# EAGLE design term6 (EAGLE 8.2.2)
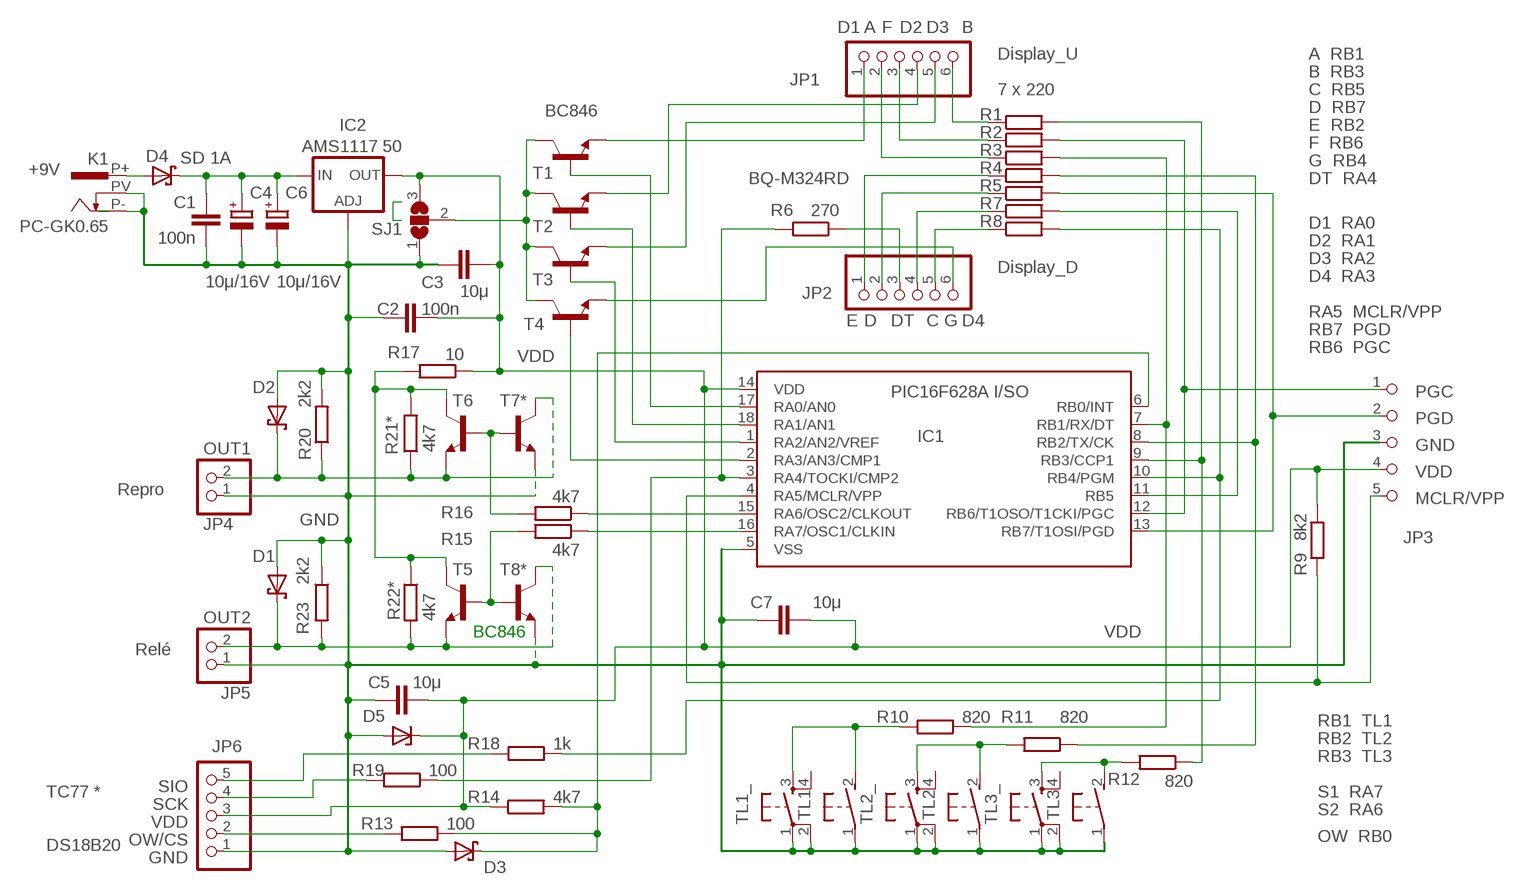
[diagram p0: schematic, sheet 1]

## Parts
C1  100n  C-EUC0805  [C0805]
C2  100n  C-EUC1206  [C1206]
C3  10μ  C-EUC1206  [C1206]
C4  10μ/16V  CPOL-EUSMCC  [SMC_C]
C5  10μ  C-EUC0805  [C0805]
C6  10μ/16V  CPOL-EUSMCD  [SMC_D]
C7  10μ  C-EUC1206  [C1206]
D1  ESD5V0S1U-02V  [SUPRES_D]
D2  ESD5V0S1U-02V  [SUPRES_D]
D3  ESD5V0S1U-02V  [SUPRES_D]
D4  SD 1A  SDIODE-1A  [SOD-5]
D5  ZENER-DIODESOD80C  [SOD80C]
IC1  PIC16F628A I/SO  PIC16F628SO  [SO-18W]
IC2  AMS1117 50  LD117AS12TR  [SOT223]
JP1  PINHD-1X061X06G  [1X06G]
JP2  PINHD-1X061X06G  [1X06G]
JP3  PIN5  [PIN5]
JP4  OUT1  PINHD-1X02_2.54-S  [1X02-S]
JP5  OUT2  PINHD-1X02_2.54-S  [1X02-S]
JP6  PINHD-1X05_2.54-S  [1X05-S]
K1  PC-GK0.65  [PC-GK0.65]
R1  R-EU_R0805  [R0805]
R2  R-EU_R0805  [R0805]
R3  R-EU_R0805  [R0805]
R4  R-EU_R0805  [R0805]
R5  R-EU_R0805  [R0805]
R6  270  R-EU_R0805  [R0805]
R7  R-EU_R0805  [R0805]
R8  R-EU_R0805  [R0805]
R9  8k2  R-EU_R0805  [R0805]
R10  820  R-EU_R0805  [R0805]
R11  820  R-EU_R0805  [R0805]
R12  820  R-EU_R0805  [R0805]
R13  100  R-EU_R0805  [R0805]
R14  4k7  R-EU_R0805  [R0805]
R15  4k7  R-EU_R0805  [R0805]
R16  4k7  R-EU_R0805  [R0805]
R17  10  R-EU_R0805  [R0805]
R18  1k  R-EU_R0805  [R0805]
R19  100  R-EU_R0805  [R0805]
R20  2k2  R-EU_R0805  [R0805]
R21*  4k7  R-EU_R0805  [R0805]
R22*  4k7  R-EU_R0805  [R0805]
R23  2k2  R-EU_R0805  [R0805]
SJ1  SJ2W  [SJ_2]
T1  BC846ASMD  [SOT23]
T2  BC817-16SMD  [SOT23-BEC]
T3  BC817-16SMD  [SOT23-BEC]
T4  BC846  BC817-16SMD  [SOT23-BEC]
T5  BC846  BC817-16SMD  [SOT23-BEC]
T6  BC846  BC817-16SMD  [SOT23-BEC]
T7*  BC846  BC817-16SMD  [SOT23-BEC]
T8*  BC846  BC817-16SMD  [SOT23-BEC]
TL1  DTSM-3  [DTSM-3]
TL1_  T_SWITCH  [T_SWITCH]
TL2  DTSM-3  [DTSM-3]
TL2_  T_SWITCH  [T_SWITCH]
TL3  DTSM-3  [DTSM-3]
TL3_  T_SWITCH  [T_SWITCH]

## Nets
A: JP1.2 R3.1
B: JP1.6 R1.1
C: JP2.4 R7.1
D: JP2.2 R5.1
D1: JP1.1 T1.2(E)
D2: JP1.4 T2.E
D3: JP1.5 T3.E
D4: JP2.6 T4.E
DT: JP2.3 R6.1
E: JP2.1 R4.1
F: JP1.3 R2.1
G: JP2.5 R8.1
GND: C1.1 C2.2 C3.2 C4.- C5.2 C6.- C7.2 D1.A D2.A D3.A D5.A IC1.5(VSS) IC2.1(ADJ) JP3.3(_3) JP4.1 JP5.1 JP6.1 K1.P- K1.PV R20.2 R23.1 SJ1.1 T7*.E T8*.E TL1.1 TL1_.1 TL1_.2 TL2.1 TL2_.1 TL2_.2 TL3.1 TL3_.1 TL3_.2
MCLR/VPP: IC1.4(RA5/MCLR/VPP) JP3.5(_5) R9.2
N$1: JP6.4 R19.2
N$2: R15.2 T5.B T8*.B
N$4: IC1.17(RA0/AN0) T1.1(B)
N$5: IC1.18(RA1/AN1) T2.B
N$6: IC1.1(RA2/AN2/VREF) T3.B
N$7: IC1.2(RA3/AN3/CMP1) T4.B
N$8: R12.2 TL3.2 TL3_.3
N$9: D1.C JP5.2 R22*.2 R23.2 T5.E T8*.C
N$10: D4.A K1.P+
N$11: D3.C IC1.6(RB0/INT) R13.1 R14.2
N$12: R16.2 T6.B T7*.B
N$13: R17.2 R21*.2 R22*.1 T5.C T6.C
N$14: JP6.5 R18.2
N$15: SJ1.2 T1.3(C) T2.C T3.C T4.C
N$17: IC1.8(RB2/TX/CK) R4.2 R11.1
N$19: IC1.11(RB5) R7.2
N$20: IC1.10(RB4/PGM) R8.2 R18.1
N$21: IC1.9(RB3/CCP1) R1.2 R12.1
N$22: IC1.3(RA4/TOCKI/CMP2) R6.2 R19.1
N$23: IC1.7(RB1/RX/DT) R3.2 R10.1
N$25: C1.2 C4.+ C6.+ D4.C IC2.3(IN)
N$28: R11.2 TL2.2 TL2_.3
N$29: R10.2 TL1.2 TL1_.3
N$34: IC1.16(RA7/OSC1/CLKIN) R15.1
N$35: IC1.15(RA6/OSC2/CLKOUT) R16.1
OW/CS: JP6.2 R13.2
PGC: IC1.12(RB6/T1OSO/T1CKI/PGC) JP3.1(_1) R2.2
PGD: IC1.13(RB7/T1OSI/PGD) JP3.2(_2) R5.2
S2: D2.C JP4.2 R20.1 R21*.1 T6.E T7*.C
VDD: C2.1 C3.1 C5.1 C7.1 D5.C IC1.14(VDD) IC2.2(OUT) IC2.4(OUT) JP3.4(_4) JP6.3 R9.1 R14.1 R17.1 SJ1.3
Unconnected: TL1_.4 TL2_.4 TL3_.4

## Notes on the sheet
- Display_U | A  RB1
- B  RB3
- 7 x 220 | C  RB5
- D  RB7
- E  RB2
- F  RB6
- G  RB4
- +9V
- BQ-M324RD | DT  RA4
- D1  RA0
- D2  RA1
- D3  RA2
- Display_D
- D4  RA3
- RA5  MCLR/VPP
- RB7  PGD
- RB6  PGC
- Repro
- JP3
- BC846
- Relé
- RB1  TL1
- RB2  TL2
- RB3  TL3
- SIO
- TC77 * | SCK | S1  RA7
- S2  RA6
- OW  RB0
- DS18B20

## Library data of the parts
C1-C3 C5 C7 = rcl:C-EU: CAPACITOR, European symbol
C4 C6 = rcl:CPOL-EU: POLARIZED CAPACITOR, European symbol
D1-D3 = pdk1:ESD5V0S1U-02V
D4 = pdk1:SDIODE-1A
D5 = diode:ZENER-DIODE: Z-Diode
IC1 = microchip:PIC16F62*: FLASH-Based 8-Bit CMOS Microcontroller Source: http://ww1.microchip.com/downloads/en/DeviceDoc/40300C.pdf; MF: MICROCHIP; MPN: PIC16F628-20I/SO; OC_FARNELL: 9760415; OC_NEWARK: 23C4986
IC2 = v-reg:LD117A?*: Low drop fixed and adjustable positive voltage regulators 1 A Source: http://www.st.com/stonline/products/literature/ds/7194/ld1117axx.pdf
JP1 JP2 = pinhead-2:PINHD-1X06: PIN HEADER
JP3 = pdk1:PIN5
JP4 JP5 = pinhead-2:PINHD-1X02: PIN HEADER
JP6 = pinhead-2:PINHD-1X05: PIN HEADER
K1 = pdk1:PC-GK0.65
R1-R20 R21* R22* R23 = rcl:R-EU_: RESISTOR, European symbol
SJ1 = jumper:SJ2W: SMD solder JUMPER
T1 = transistor-npn:BC846*: NPN Transistor
T2-T6 T7* T8* = transistor-npn:BC817*: NPN Transistor
TL1-TL3 = switch-tact_1:DTSM-3
TL1_ TL2_ TL3_ = pdk1:T_SWITCH

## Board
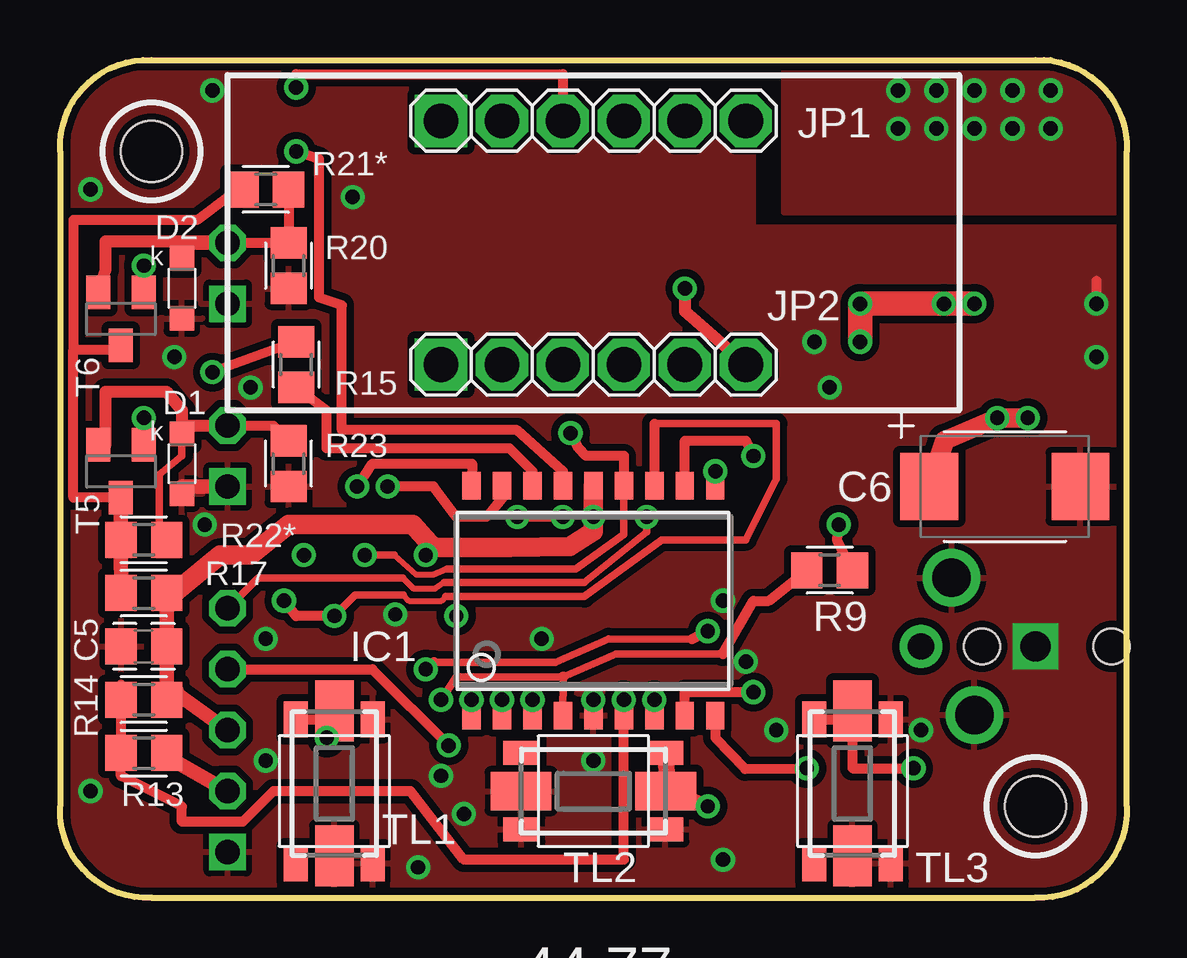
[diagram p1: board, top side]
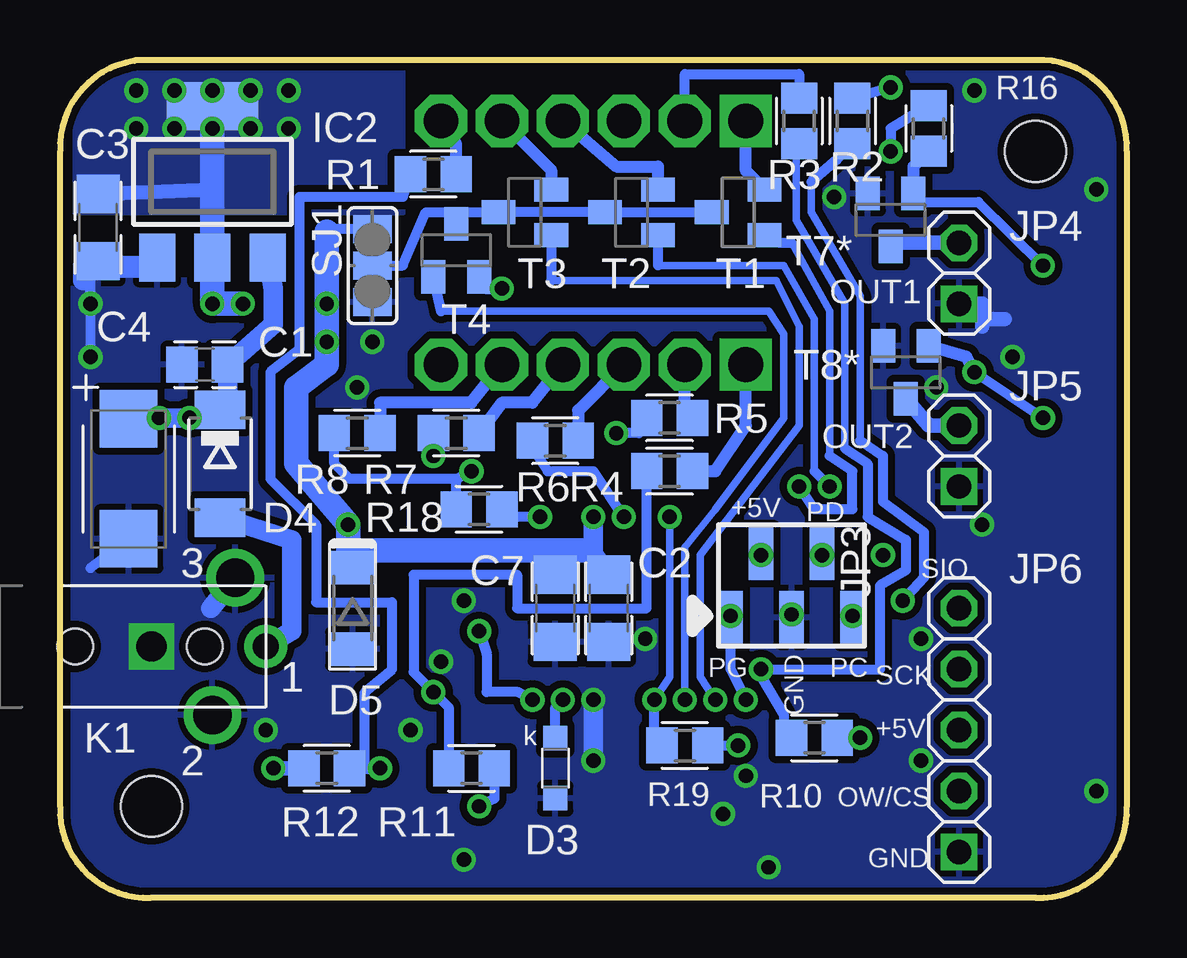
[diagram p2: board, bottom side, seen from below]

Size 44.45 x 34.92 mm. Coordinates in mm from the lower left corner, seen from the top.
Outline: 40.64,34.92 arc-95 44.45,31.11 44.45,3.81 arc-95 40.64,0 3.81,0 arc-95 0,3.81 0,31.11 arc-95 3.81,34.92 41.27,34.92
Copper layers (1*16): Top 0.035mm / dielectric 1.5mm / Bottom 0.035mm
Design rules "default *": minimum track width 6mil, minimum drill 0.35mm, track to track 6mil, track to pad 6mil, pad to pad 6mil, via to via 6mil, smd to smd 0mil, copper to edge 5mil, drill to drill 6mil, minimum pad ring 10mil, minimum via ring 8mil, stop-mask expansion 4mil, vias tented up to drill 0mil, thermal gap 10mil
Holes 2.54 mm at 40.64,3.81 3.81,31.11

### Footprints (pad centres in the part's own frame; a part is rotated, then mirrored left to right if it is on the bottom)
C0805 = smd 1.3 x 1.5: 1 -0.95,0; 2 0.95,0
C1206 = smd 1.6 x 1.8: 1 -1.4,0; 2 1.4,0
SMC_C = smd 2.4 x 2.4: + -2.5,0; - 2.5,0
SMC_D = smd 2.4 x 2.8: + -3.15,0; - 3.15,0
SUPRES_D = smd 1.016 x 1.016: A 1.25,0; C -1.25,0
SOD-5 = smd 1.6 x 2.1: A 2.25,0; C -2.25,0
SOD80C = smd 1.4 x 1.8: A 1.7,0; C -1.7,0
SO-18W = smd 0.762 x 1.143: 1 -5.08,-4.788; 2 -3.81,-4.788; 3 -2.54,-4.788; 4 -1.27,-4.788; 5 0,-4.788; 6 1.27,-4.788; 7 2.54,-4.788; 8 3.81,-4.788; 9 5.08,-4.788; 10 5.08,4.788; 11 3.81,4.788; 12 2.54,4.788; 13 1.27,4.788; 14 0,4.788; 15 -1.27,4.788; 16 -2.54,4.788; 17 -3.81,4.788; 18 -5.08,4.788
SOT223 = smd 1.5 x 2: 1 -2.3,-3.15; 2 0,-3.15; 3 2.3,-3.15 | smd 3.8 x 2: 4 0,3.15
1X06G = drill 1.448 pad 1.93 square: 1 -6.35,0 | drill 1.448 pad 1.93 octagon: 2 -3.81,0; 3 -1.27,0; 4 1.27,0; 5 3.81,0; 6 6.35,0
PIN5 = smd 1.016 x 2.2: 1 -1.905,1.33; 2 -0.635,-1.33; 3 0.635,1.33; 4 1.905,-1.33; 5 3.175,1.33
1X02-S = drill 1.016 square: 1 -1.27,0 | drill 1.016 octagon: 2 1.27,0
1X05-S = drill 1.016 square: 1 -5.08,0 | drill 1.016 octagon: 2 -2.54,0; 3 0,0; 4 2.54,0; 5 5.08,0
PC-GK0.65 = drill 1.1 pad 1.778: P+ -5.08,0 | drill 1.6: P- -2.857,2.857; PV -3.81,-2.857 | hole 1.5: -2.54,0; 2.857,0
R0805 = smd 1.3 x 1.5: 1 -0.95,0; 2 0.95,0
SJ_2 = smd 1.168 x 1.6: 1 -1.524,0; 2 0,0; 3 1.524,0
SOT23 = smd 1 x 1.4: 1 -0.95,-1.1; 2 0.95,-1.1; 3 0,1.1
SOT23-BEC = smd 1 x 1.4: B -0.95,-1.1; C 0,1.1; E 0.95,-1.1
DTSM-3 = smd 2.54 x 1.6: 1 -3.018,0; 2 3.018,0
T_SWITCH = smd 1.5 x 1: 1 -3,1.6; 2 3,1.6; 3 -3,-1.6; 4 3,-1.6

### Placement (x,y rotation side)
C1  38.42,22.23 0 bottom
C2  21.59,12.06 270 bottom
C3  42.86,27.94 270 bottom
C4  41.59,17.46 270 bottom
C5  3.49,10.48 180 top
C6  39.37,17.14 0 top
C7  23.81,12.06 270 bottom
D1  5.08,18.1 270 top
D2  5.08,25.4 270 top
D3  23.81,5.4 270 bottom
D4  37.78,18.1 270 bottom
D5  32.26,12.06 270 bottom
IC1  22.23,12.38 0 top
IC2  38.1,29.84 0 bottom
JP1  22.23,32.38 0 top
JP2  22.23,22.23 0 top
JP3  13.34,13.02 180 bottom
JP4  6.99,26.04 90 bottom
JP5  6.99,18.41 90 bottom
JP6  6.99,6.99 90 bottom
K1  40.96,10.48 180 bottom
R1  28.89,30.16 180 bottom
R2  11.43,32.38 270 bottom
R3  13.65,32.38 270 bottom
R4  19.05,17.78 180 bottom
R5  19.05,20 180 bottom
R6  23.81,19.05 180 bottom
R7  27.94,19.37 180 bottom
R8  32.07,19.37 180 bottom
R9  32.07,13.65 180 top
R10  13.02,6.67 0 bottom
R11  27.3,5.4 0 bottom
R12  33.34,5.4 180 bottom
R13  3.49,6.03 0 top
R14  3.49,8.26 180 top
R15  9.84,22.23 90 top
R16  8.26,32.07 270 bottom
R17  3.49,12.7 180 top
R18  26.99,16.19 0 bottom
R19  18.41,6.35 0 bottom
R20  9.53,26.35 270 top
R21*  8.57,29.53 180 top
R22*  3.49,14.92 0 top
R23  9.53,18.1 90 top
SJ1  31.43,26.35 90 bottom
T1  16.19,28.57 90 bottom
T2  20.64,28.57 90 bottom
T3  25.08,28.57 90 bottom
T4  27.94,26.99 0 bottom
T5  2.54,17.78 180 top
T6  2.54,24.13 180 top
T7*  9.84,28.26 180 bottom
T8*  9.21,21.91 180 bottom
TL1  11.43,4.76 90 top
TL1_  11.43,4.45 270 top
TL2  22.23,4.45 0 top
TL2_  22.23,4.45 180 top
TL3  33.02,4.76 90 top
TL3_  33.02,4.45 270 top

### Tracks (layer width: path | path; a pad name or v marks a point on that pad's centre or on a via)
A
  Bottom 0.406: JP1.2 18.41,34.34 13.65,34.34 R3.1
B
  Bottom 0.508: R1.1 27.94,31.43 JP1.6
C
  Bottom 0.508: JP2.4 24.77,20.64 26.04,20.64 R7.1
D
  Bottom 0.406: R5.1 18.41,20.32
  Bottom 0.508: 18.41,20.32 JP2.2
D1
  Bottom 0.508: T1.2 15.88,30.31 JP1.1
D2
  Bottom 0.508: JP1.4 21.27,30.48 19.54,30.48 T2.E
D3
  Bottom 0.508: JP1.5 23.98,30.33 T3.E
D4  (via drill 0.6)
  Top 0.508: JP2.6 26.04,24.45 v26.04,25.4
  Bottom 0.508: v26.04,25.4 26.67,25.4 T4.E
DT
  Bottom 0.406: 22.86,19.37 R6.1
  Bottom 0.508: JP2.3 22.86,20.32 22.86,19.37
E
  Bottom 0.508: R4.1 17.14,17.78 15.88,19.68 JP2.1
F  (via drill 0.6)
  Top 0.406: JP1.3 20.95,34.34 9.84,34.34 9.84,34.29 v9.84,33.78
  Bottom 0.406: R2.1 v9.84,33.78
G
  Bottom 0.406: R8.1
  Bottom 0.508: JP2.5 27.3,20.64 31.11,20.64 R8.1
GND  (via drill 0.6, 1.27)
  Top 0.406: 43.18,25.72 v43.18,24.77
  Top 0.61: JP5.1 5.1,17.14
  Bottom 0.406: IC2.1 40.4,26.04 43.18,26.04 v43.18,24.77 | v43.18,24.77 v43.18,22.54 | 43.18,13.74 C4.- | v43.18,24.77 43.18,26.36 C3.2
  Bottom 0.61: JP4.1 6.03,24.77 6.03,23.81 | 5.08,24.13 5.71,24.13
  Bottom 0.813: 42.55,26.35 40.32,26.35 | C3.2 42.55,26.35 | 42.55,26.35 43.5,26.35 43.5,25.72 | v22.23,5.71 v22.23,8.26 | K1.PV 38.17,12.06
  other vias: 28.57,9.84 27.62,12.38 35.88,6.99 12.19,29.21 27.62,1.59 14.92,1.27 29.84,6.99 15.88,5.08 8.57,10.79 1.27,4.45 16.83,3.49 13.97,11.81 8.57,5.71 40.64,10.48 7.94,21.27 4.76,22.54 6.35,33.66 31.43,23.18 6.03,15.56 20.07,10.79 32.07,21.27 1.27,29.53
  pour Bottom (isolate 0.305): 0,0 0,34.92 28.57,34.92 28.57,25.72 44.45,25.72 44.45,0
  pour Top (isolate 0.305): 28.89,34.92 0,34.92 0,0 44.45,0 44.45,27.94 28.89,27.94
MCLR/VPP  (via drill 0.6)
  Top 0.305: 27.62,10.16 23.18,10.16 20.97,9.22 IC1.4 | 20.95,9.21 16.51,9.21 v15.88,8.26
  Top 0.406: 27.62,10.16 28.89,12.38 29.53,12.38 R9.2 | 20.97,9.22 20.95,9.21
  Bottom 0.305: JP3.5 v16.51,11.75
  Bottom 0.406: JP3.5 16.51,9.53 v15.88,8.26
N$1  (via drill 0.6)
  Top 0.406: JP6.4 13.02,9.53 v16.19,6.35
  Bottom 0.406: R19.2 v16.19,6.35
N$2  (via drill 0.6)
  Top 0.406: R15.2 v6.35,21.91
  Top 0.508: v3.49,20 T5.B
  Bottom 0.406: v3.49,20 v6.35,21.91
  Bottom 0.508: v6.35,21.91 6.67,22.54 T8*.B
N$4  (via drill 0.6)
  Top 0.406: IC1.17 18.41,16.64 17.78,15.88 16.51,15.88 15.56,17.14 v13.65,17.14
  Bottom 0.305: 12.38,18.41 12.38,24.45 13.97,27.3
  Bottom 0.406: 12.38,18.41 11.43,17.78 11.43,16.19 13.02,16.19 v13.65,17.14 | T1.1 14.48,27.31 13.97,27.3
N$5  (via drill 0.6)
  Top 0.406: v12.38,17.14 13.02,18.1 17.17,18.1 17.14,16.83 IC1.18
  Bottom 0.305: 13.02,17.78 13.02,24.13 14.29,26.35 19.54,26.35
  Bottom 0.406: v12.38,17.14 13.02,17.78 | T2.B 19.54,26.35
N$6  (via drill 0.6)
  Top 0.406: IC1.1 v17.14,8.26
  Bottom 0.305: v17.14,8.26 17.78,9.21 17.78,14.29 13.65,19.68 13.65,23.81 14.61,25.72 23.98,25.72
  Bottom 0.406: T3.B 23.98,25.72
N$7  (via drill 0.6)
  Top 0.406: IC1.2 v18.41,8.26
  Bottom 0.305: v18.41,8.26 18.41,14.61 17.14,16.19 14.29,20 14.29,23.5 14.92,24.45 28.57,24.45
  Bottom 0.406: 28.57,24.45 T4.B
N$8  (via drill 0.6)
  Top 0.406: TL3_.3 33.02,7.45 TL3.2 33.02,5.4 v35.56,5.4
  Bottom 0.61: v35.56,5.4 R12.2
N$9
  Top 0.305: D1.C 5.08,18.41 4.13,17.65 4.13,15.56
  Top 0.406: 4.13,15.56 4.12,15.56 R22*.2 | JP5.2 8.89,19.68 R23.2
  Top 0.508: T5.E 1.91,18.88 1.91,21.08 4.45,21.08 5.08,20.32 5.08,19.68 | 5.08,19.68 D1.C | 5.08,19.68 JP5.2
  Bottom 0.61: JP5.2 8.26,19.68 T8*.C
N$10
  Bottom 0.61: 37.78,15.88 D4.A
  Bottom 0.813: 37.78,15.88 34.8,14.92 34.8,11.11 K1.P+
N$11  (via drill 0.6)
  Top 0.406: 2.54,8.89 R14.2 R13.1 2.54,5.08 5.08,3.81 5.08,3.17 7.62,3.17 8.89,4.45 14.61,4.45 16.83,1.59 23.5,1.59 IC1.6 v23.5,8.26
  Bottom 0.406: D3.C 23.81,7.94 v23.5,8.26
N$12  (via drill 0.6)
  Top 0.508: T6.B v3.5,26.35
  Bottom 0.406: T7*.B 8.57,29.01 6.18,29.01 v3.5,26.35
  Bottom 0.508: R16.2 8.89,30.48 T7*.B
N$13
  Top 0.406: 0.56,22.86 2.37,22.86 T6.C | T5.C 0.56,16.68 0.56,22.86 | R21*.2 6.99,29.21 5.71,28.26 0.56,28.26 0.56,22.86 | R22*.1 2.54,14.61 2.54,14.6
  Top 0.61: T5.C 2.54,14.6 R17.2
N$14  (via drill 0.6)
  Top 0.254: 16.02,13.15 15.62,12.88 14.74,12.88 14.29,13.34
  Top 0.305: v24.45,15.88 24.45,15.24 21.84,13.15 16.02,13.15 | JP6.5 8.26,13.34 14.29,13.34
  Bottom 0.406: v24.45,15.88 25.72,15.88 R18.2
N$15
  Bottom 0.406: T1.3 T2.C T3.C 27.62,28.57 | 27.62,28.57 T4.C | SJ1.2 30.16,26.35 29.21,28.57 27.62,28.57
N$16  (via drill 0.6)
  other vias: 10.16,14.29
N$17  (via drill 0.6)
  Top 0.406: IC1.8 26.04,8.57 v28.89,8.57
  Bottom 0.406: 20,14.61 R4.2 20,15.24 20,14.61 | 20,14.61 20,12.06 25.4,12.06 25.4,13.46 29.72,13.46 29.72,9.4 v28.89,8.57 28.26,7.94 R11.1
N$19  (via drill 0.6)
  Top 0.406: IC1.11 26.04,19.05 28.57,19.05 v28.89,18.41
  Bottom 0.406: R7.2 v28.89,18.42 v28.89,18.41
N$20  (via drill 0.6)
  Top 0.406: v27.3,17.78 IC1.10
  Bottom 0.406: R8.2 33.02,18.1 32.38,17.46 28.05,17.46 | 28.05,17.46 27.94,17.46 v27.3,17.78 | R18.1 27.94,17.36 28.05,17.46
N$21  (via drill 0.6)
  Top 0.406: IC1.9 27.3,6.67 28.55,5.37 v31.11,5.4
  Bottom 0.406: R1.2 30.16,29.21 34.48,29.21 34.48,22.86 35.69,21.91 35.69,17.46 33.78,15.56 33.78,12.32 30.61,12.32 30.61,9.53 31.75,8.57 31.75,5.4 | R12.1 32.07,5.39 v31.11,5.4
  Bottom 0.508: v31.11,5.4 31.75,5.4
N$22  (via drill 0.6)
  Top 0.406: v19.68,8.26 IC1.3 | v20.95,15.88 v19.05,15.88
  Bottom 0.305: v19.68,8.26 19.05,9.21 v19.05,15.88
  Bottom 0.406: R6.2 24.76,18.73 24.13,17.78 22.23,17.78 v20.95,15.88 | v19.68,8.26 19.68,6.99 19.36,6.67 R19.1
N$23  (via drill 0.6)
  Top 0.305: 26.33,10.77 22.86,10.79 20.63,9.82 15.58,9.82
  Top 0.406: IC1.7 v24.77,8.26 | v26.99,11.11 26.33,10.77 | 15.58,9.82 v15.24,9.53
  Bottom 0.305: 13.78,31.43 13.78,28.26 11.75,24.77 11.75,18.73
  Bottom 0.406: v26.99,11.11 26.67,10.16 26.67,8.57 25.38,8.57 v24.77,8.26 | R3.2 13.78,31.43 | 11.75,18.73 10.79,18.1 10.79,15.88 9.21,14.92 9.21,13.65 10.29,13.02 10.29,9.53 v15.24,9.53 15.24,9.21 14.29,7.62 14.29,6.67 R10.1
N$25  (via drill 0.6)
  Top 0.813: C6.+ 36.85,19.05 v39.05,20 v40.32,20
  Bottom 0.813: 37.47,20 C1.2 | 37.47,20 D4.C | C1.2 | C1.2 35.56,23.89 35.56,25.4 IC2.3 | 37.47,20 v39.05,20 41.27,20 C4.+
N$28  (via drill 0.6)
  Top 0.61: TL2.2 25.24,4.76 TL2_.3 | TL2_.3 25.39,4.78 | TL2_.3 25.39,4.46 v26.99,3.81
  Bottom 0.406: R11.2 26.35,4.13 v26.99,3.81
N$29  (via drill 0.6)
  Top 0.406: v11.11,6.67 11.43,6.99 TL1.2 11.43,7.45 TL1_.3
  Bottom 0.61: R10.2 v11.11,6.67
N$34
  Top 0.406: IC1.16 19.68,17.78 18.73,18.73 11.11,18.73 11.11,20.32 R15.1
N$35  (via drill 0.6)
  Top 0.406: IC1.15 20.95,17.78 19.05,19.49 11.75,19.49 11.75,24.7 10.79,25.02 10.79,30.8 v9.84,31.11
  Bottom 0.406: R16.1 9.84,32.07 v9.84,31.11
OW/CS
  Top 0.61: R13.2 4.76,5.71 JP6.2
PGC  (via drill 0.6)
  Top 0.254: 14.3,12.62 14.54,12.38 15.9,12.38 16.07,12.56
  Top 0.305: 24.77,19.76 29.84,19.76 29.84,17.46 28.57,14.92 25.08,14.92 21.84,12.56 16.07,12.56 | 14.3,12.62 12.3,12.62 v11.43,11.75
  Top 0.406: 24.77,19.76 IC1.12 | v11.43,11.75 9.84,11.75 v9.34,12.38
  Bottom 0.305: 13.14,29.84 13.14,28.57 11.11,25.08 11.11,19.05
  Bottom 0.406: R2.2 12.06,30.8 13.14,29.84 | 11.11,19.05 10.16,18.41 10.16,16.51 8.46,15.24 8.46,13.34 v9.34,12.38 | JP3.1 v11.43,11.75
PGD  (via drill 0.6)
  Top 0.254: 16.14,13.72 15.56,13.46 14.86,13.46 13.92,14.29
  Top 0.305: IC1.13 23.5,15.15 21.49,13.72 16.14,13.72 | 13.92,14.29 v12.7,14.29
  Top 0.406: v21.27,19.37 21.61,18.73 21.91,18.41 23.5,18.41 IC1.13
  Bottom 0.406: R5.2 20.32,19.37 v21.27,19.37 | JP3.2 v12.7,14.29
S2
  Top 0.406: R21*.1 R20.1 | R20.1 JP4.2 | R20.1 8.98,27.3
  Top 0.508: T6.E 1.91,26.18 1.91,27.37 5.08,27.37 5.08,27.3 D2.C
  Top 0.61: D2.C 5.06,26.97 5.08,27.3 JP4.2
  Bottom 0.406: 9.99,27.3 T7*.C
  Bottom 0.61: JP4.2 9.99,27.3
VDD  (via drill 0.6)
  Top 0.406: v15.24,14.29 15.24,15.01 14.69,15.56 | R9.1 32.38,14.92 v32.45,15.56
  Top 0.61: R14.1 C5.1 4.44,12.64 R17.1 | 4.76,8.57 JP6.3
  Top 0.813: IC1.14 v22.23,15.88 22.23,15.27 21.24,14.64 18.73,14.61 17.74,14.59 15.56,14.61 14.69,15.56 9.53,15.56 7.94,14.29 6.67,14.29 4.76,12.7 4.5,12.7 4.44,12.64 | R14.1 4.76,8.57
  Top 1.016: v33.34,23.18 v33.34,24.77 v36.83,24.77 v38.1,24.77
  Bottom 0.305: C7.1 24.2,14.48
  Bottom 0.406: D5.C 32.38,14.1 32.45,14.48 | JP3.4 v15.24,14.29 | SJ1.3 33.34,27.88 33.34,27.77
  Bottom 0.61: C3.1 38.1,29.52 | 22.23,14.35 22.36,14.48
  Bottom 0.813: C2.1 22.23,14.35 v22.23,15.88 22.23,15.9
  Bottom 1.016: IC2.4 38.1,29.52 IC2.2 v38.1,24.77 v36.83,24.77 | 22.36,14.48 24.2,14.48 32.45,14.48 v32.45,15.56 34.61,18.1 34.61,21.27 33.34,22.23 v33.34,24.77 v33.34,23.18 33.34,27.77
  other vias: 36.51,32.07 39.69,33.66 36.51,33.66 39.69,32.07 38.1,33.66 38.1,32.07 34.92,33.66 34.92,32.07 41.27,33.66 41.27,32.07
  pour Bottom (isolate 0.305, no thermals): 43.81,28.57 30.16,28.57 30.16,34.92 43.81,34.92
  pour Top (isolate 0.305, no thermals): 30.16,34.92 30.16,28.57 44.45,28.57 44.45,34.92

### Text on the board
bNames: OUT1 | OUT2 | PD | +5V | SIO | GND | SCK | PC | PG | +5V | OW/CS | GND
bDocu: k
